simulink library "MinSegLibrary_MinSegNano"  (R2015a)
settings: Solver=ode45  StartTime=0.0  StopTime=10.0  RelTol=1e-3
undefined symbols (not defined in the file or in its folder): Vsupply
libraries: arduinolib x2, simulink x1

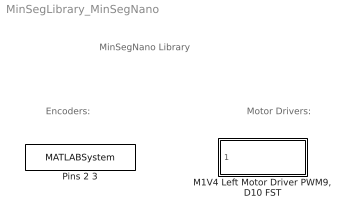
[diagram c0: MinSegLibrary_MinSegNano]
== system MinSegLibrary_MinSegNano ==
  note: Motor Drivers:
  note: Encoders:
  note: MinSegNano Library
  "M1V4 Left Motor Driver PWM9, D10 FST" : Subsystem
  Pins 2 3 : MATLABSystem  System=Encoder_arduino_uno_nano  Encoder=0  PinA=2  PinB=3

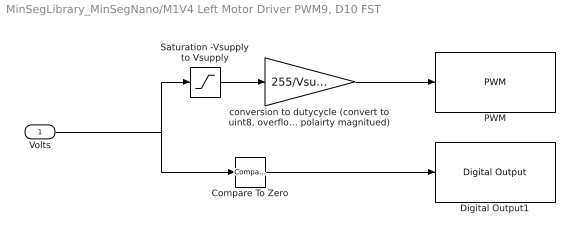
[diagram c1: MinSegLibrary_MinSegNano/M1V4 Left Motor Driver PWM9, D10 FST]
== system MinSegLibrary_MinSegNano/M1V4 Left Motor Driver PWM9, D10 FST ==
  Volts : Inport
  Compare To Zero : simulink/Logic and Bit Operations/Compare To Zero  relop=<  OutDataTypeStr=boolean
  Digital Output1 : arduinolib/Digital Output  pinNumber=10  blockPlatform=arduino
  PWM : arduinolib/PWM  pinNumber=9  blockPlatform=arduino
  Saturation -Vsupply to Vsupply : Saturate  UpperLimit=Vsupply  LowerLimit=-Vsupply  OutDataTypeStr=single
  "conversion to dutycycle (convert to uint8, overflow will provide reverse polairty magnitued)" : Gain  Gain=255/Vsupply  OutDataTypeStr=uint8
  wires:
  Volts/1 -> Compare To Zero/1, Saturation -Vsupply to Vsupply/1
  Saturation -Vsupply to Vsupply/1 -> "conversion to dutycycle (convert to uint8, overflow will provide reverse polairty magnitued)"/1
  "conversion to dutycycle (convert to uint8, overflow will provide reverse polairty magnitued)"/1 -> PWM/1
  Compare To Zero/1 -> Digital Output1/1
